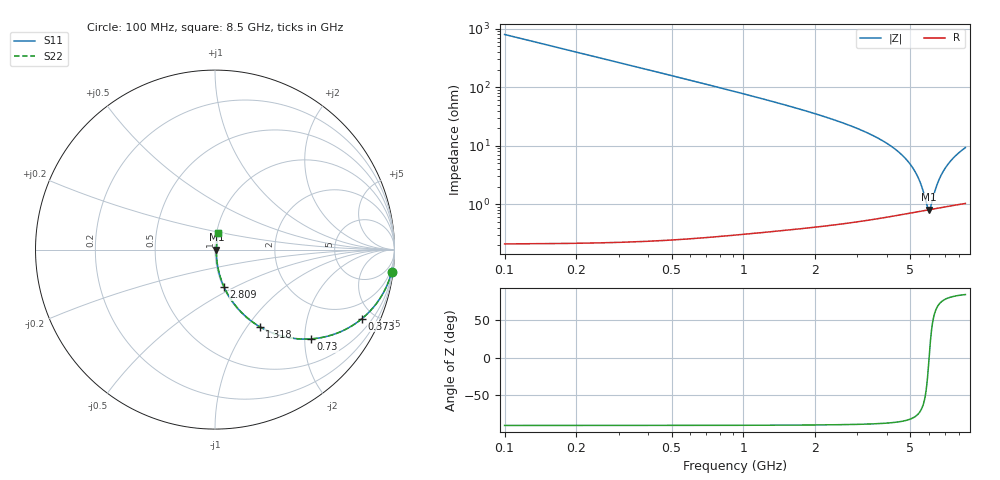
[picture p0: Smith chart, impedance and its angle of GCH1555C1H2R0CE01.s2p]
!Murata Part Number: GCH1555C1H2R0CE01
!These Parameters are Measured in Series Mode Connection
!Data Generated on Mar 13, 2026
!  o--ll--o
!Port1  Port2
!  o------o
!Operation Temp=25[degC], DC Bias Voltage=0[V]
!Freq. Start=100[MHz] Stop=9[GHz] 401[Steps]
# Hz S RI R 50
!Freq.(Hz) S11(Real) S11(Imag) S21(Real) S21(Imag) S12(Real) S12(Imag) S22(Real) S22(Imag)
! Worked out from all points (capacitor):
!   401 points, 100 MHz to 8.5 GHz, reference 50 ohm
!   read as one part in series: C = 2 pF near 142 MHz
!   lowest |Z| = 811 mohm at 5.98 GHz (marker M1)
!   series resonance near 5.991 GHz, so ESL is about 350 pH
!   S11 on the Smith chart (normalised r, x): 100 MHz: 1, -16; 373 MHz: 1.00, -4.25; 730 MHz: 1.01, -2.15; 1.318 GHz: 1.01, -1.15; 2.809 GHz: 1.01, -0.44; 8.5 GHz: 1.02, +0.18
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1e8  0.9844 -0.1237  0.0156 0.1237  0.0156 0.1237  0.9844 -0.1237
2.26e8  0.925 -0.2631  0.075 0.2631  0.075 0.2631  0.925 -0.2631
3.73e8  0.8184 -0.385  0.1816 0.385  0.1816 0.385  0.8184 -0.385
7.3e8  0.535 -0.4975  0.465 0.4975  0.465 0.4975  0.535 -0.4975
1.003e9  0.3726 -0.4815  0.6274 0.4815  0.6274 0.4815  0.3726 -0.4815
1.318e9  0.2486 -0.4292  0.7514 0.4292  0.7514 0.4292  0.2486 -0.4292
1.507e9  0.1974 -0.3944  0.8026 0.3944  0.8026 0.3944  0.1974 -0.3944
2.053e9  0.1069 -0.303  0.8931 0.303  0.8931 0.303  0.1069 -0.303
2.809e9  0.0502 -0.2076  0.9498 0.2076  0.9498 0.2076  0.0502 -0.2076
2.914e9  0.0454 -0.1967  0.9546 0.1967  0.9546 0.1967  0.0454 -0.1967
4.3e9  0.014 -0.0869  0.986 0.0869  0.986 0.0869  0.014 -0.0869
5.161e9  0.00871 -0.0386  0.9913 0.0386  0.9913 0.0386  0.00871 -0.0386
5.455e9  0.0081 -0.0242  0.9919 0.0242  0.9919 0.0242  0.0081 -0.0242
5.707e9  0.00792 -0.0125  0.9921 0.0125  0.9921 0.0125  0.00792 -0.0125
5.896e9  0.00797 -0.00411  0.992 0.00411  0.992 0.00411  0.00797 -0.00411
5.98e9  0.00804 -0.000471  0.992 0.000471  0.992 0.000471  0.00804 -0.000471
6.085e9  0.00815 0.004  0.9918 -0.004  0.9918 -0.004  0.00815 0.004
6.337e9  0.00859 0.0144  0.9914 -0.0144  0.9914 -0.0144  0.00859 0.0144
6.547e9  0.0091 0.0227  0.9909 -0.0227  0.9909 -0.0227  0.0091 0.0227
7.114e9  0.0111 0.044  0.9889 -0.044  0.9889 -0.044  0.0111 0.044
7.723e9  0.0139 0.065  0.9861 -0.065  0.9861 -0.065  0.0139 0.065
8.5e9  0.0185 0.0898  0.9815 -0.0898  0.9815 -0.0898  0.0185 0.0898
